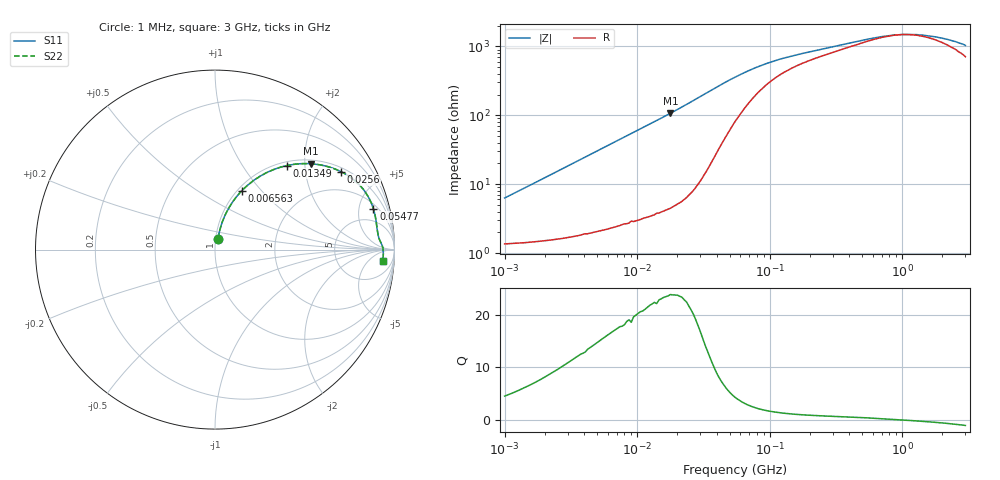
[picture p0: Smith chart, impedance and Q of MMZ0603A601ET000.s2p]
! S-Parameter Data Generated by TDK Corporation
! Copyright(C) 2025 TDK Corporation.
! All Rights Reserved.
! TDK P/N: MMZ0603A601ET000 (Chip Bead)
! Property: |Z|=600ohm at 100MHz
! Size(LxWxT): 0.6x0.3x0.3mm
! Model Type: s2p (Touchstone File Format Version 1.0)
! Frequency: DC=Yes Start=1MHz Stop=3000MHz 202points Log-sweep
! Model Generated on Feb. 6, 2025
! Terms and conditions regarding TDK Simulation Models:
! 1)This simulation model is being provided solely for informational
!  purposes. Please refer to the specifications of the products in
!  terms of detailed characteristics of such products.
! 2)In no event shall TDK Corporation of any of its subsidiaries be
!  liable for any loss or damage arising, directly or indirectly,
!  from any information contained in this simulation model, including,
!  but not limited to loss or damages arising from any inaccuracies,
!  omissions or errors in connection with such information.
! 3)Any and all copyrights on this simulation model are owned by
!  TDK Corporation.  Duplication or redistribution of this simulation
!  model without prior written permission from TDK Corporation
!  is prohibited.
! 4)This simulation model is subject to any modification or change
!  without any prior notice.
! 5)Neither TDK Corporation nor any of its subsidiaries shall make any
!  warranty, express or implied, including but not limited to the
!  correctness, implied warranties of merchantability and fitness for
!  a particular purpose with respect to this simulation models.
! 6)The use of this simulation model shall be deemed to have consented
!  to the terms and conditions hereof.
! Port Assignments:
!  1 ---@@@--- 2
! Applicable Conditions:
!  Temperature = 25 degC
!  DC Bias Current = 0 A
!  Small Signal Operation
# Hz S MA R 50
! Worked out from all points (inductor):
!   201 points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, 1 MHz to 3 GHz, reference 50 ohm
!   read as one part in series: L = 979 nH near 1.041 MHz
!   highest Q = 23.8 at 17.86 MHz (marker M1), where L = 956 nH
!   self-resonance near 984.3 MHz
!   S11 on the Smith chart (normalised r, x): 1 MHz: 1.03, +0.12; 6.563 MHz: 1.05, +0.79; 13.49 MHz: 1.07, +1.61; 25.6 MHz: 1.15, +3.14; 54.77 MHz: 2.62, +6.97; 3 GHz: 15, -15
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1000000  0.06204 74.1  0.9848 -3.5  0.9848 -3.5  0.06204 74.1
2055611  0.1241 76.1  0.9775 -7.1  0.9775 -7.1  0.1241 76.1
3900413  0.228 72.4  0.9559 -13.1  0.9559 -13.1  0.228 72.4
6563319  0.3613 65.5  0.9113 -21.1  0.9113 -21.1  0.3613 65.5
9410094  0.4812 58.4  0.8525 -28.7  0.8525 -28.7  0.4812 58.4
1.349163e7  0.615 49.5  0.7616 -37.9  0.7616 -37.9  0.615 49.5
1.461624e7  0.6446 47.4  0.7369 -40.1  0.7369 -40.1  0.6446 47.4
1.785516e7  0.7167 41.9  0.668 -45.7  0.668 -45.7  0.7167 41.9
2.559965e7  0.8262 31.6  0.5253 -55.6  0.5253 -55.6  0.8262 31.6
3.127247e7  0.8689 26.2  0.4422 -60.1  0.4422 -60.1  0.8689 26.2
3.670325e7  0.8914 22.2  0.3794 -62.6  0.3794 -62.6  0.8914 22.2
5.477226e7  0.9112 14.4  0.2547 -62.6  0.2547 -62.6  0.9112 14.4
7.852918e7  0.9115 9.7  0.1848 -56.6  0.1848 -56.6  0.9115 9.7
9.984923e7  0.9106 7.7  0.1556 -51.2  0.1556 -51.2  0.9106 7.7
1.431579e8  0.9119 5.5  0.127 -43.4  0.127 -43.4  0.9119 5.5
2.136344e8  0.9159 3.9  0.1068 -36.1  0.1068 -36.1  0.9159 3.9
5.583748e8  0.9315 1.4  0.07262 -18.7  0.07262 -18.7  0.9315 1.4
8.005644e8  0.9356 0.5  0.06505 -7.6  0.06505 -7.6  0.9356 0.5
1.017911e9  0.9372 -0.1  0.06278 1.4  0.06278 1.4  0.9372 -0.1
1.519029e9  0.9381 -1.2  0.06497 17.1  0.06497 17.1  0.9381 -1.2
2.177892e9  0.9379 -2.4  0.0737 31.5  0.0737 31.5  0.9379 -2.4
3e9  0.936 -3.8  0.09034 43.0  0.09034 43.0  0.936 -3.8
